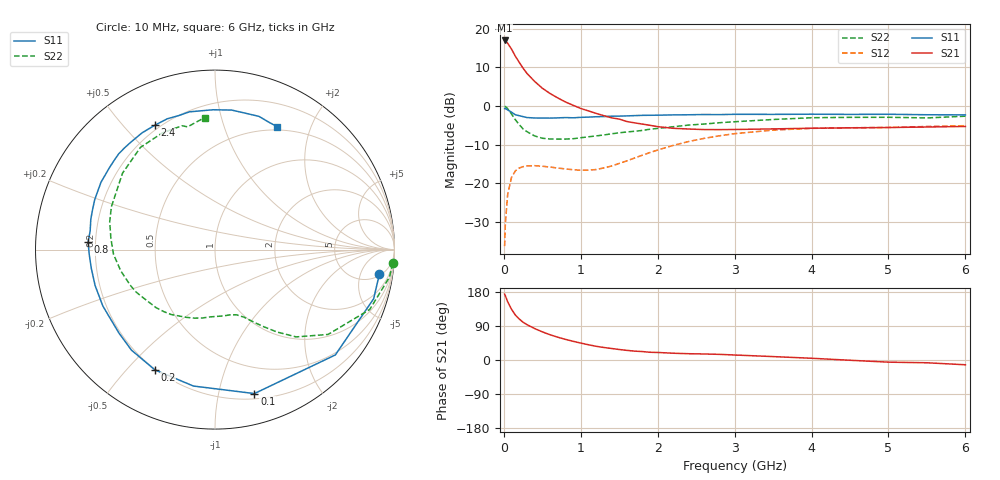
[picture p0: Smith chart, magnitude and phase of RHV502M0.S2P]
! SIEMENS Small Signal Semiconductors
! BFR106
! Si NPN RF Bipolar Junction Transistor in SOT23
! VCE = 0.5 V  IC = 2 mA
! Common Emitter S-Parameters:  August  1996
# GHz  S  MA  R  50
!  f  S11  S21  S12  S22
! GHz  MAG  ANG  MAG  ANG  MAG  ANG  MAG  ANG
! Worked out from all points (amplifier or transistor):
!   36 points, 10 MHz to 6 GHz, reference 50 ohm
!   highest |S21| = 17.0 dB at 10 MHz (marker M1)
!   |S21| within 3 dB of that: start of sweep to 120.3 MHz
!   unconditionally stable (mu >= 1): 737.2 MHz to end of sweep
!   at 250 MHz: K = 0.35, MSG = 12.8 dB, |S12| = -15.7 dB
!   at 1.4 GHz: K = 1.40, MAG = 2.5 dB, |S12| = -15.6 dB
!   at 6 GHz: K = 1.03, MAG = -1.1 dB, |S12| = -5.1 dB
!   S11 on the Smith chart (normalised r, x): 10 MHz: 5, -11; 100 MHz: 0.25, -1.28; 200 MHz: 0.20, -0.60; 800 MHz: 0.17, +0.03; 2.4 GHz: 0.18, +0.61; 6 GHz: 0.46, +1.53
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0.01  0.9259 -8.6  7.087 173.9  0.0152 85.9  0.9929 -4.4
0.02  0.9253 -17.2  6.999 169.3  0.0302 82.7  0.9839 -9.0
0.05  0.891 -41.2  6.503 153.5  0.0716 66.5  0.9242 -21.2
0.1  0.8316 -74.7  5.468 133.9  0.1189 49.7  0.7874 -36.9
0.15  0.7696 -99.0  4.422 118.6  0.144 37.6  0.664 -47.1
0.2  0.749 -116.6  3.688 108.2  0.157 30.3  0.5738 -53.1
0.25  0.7283 -129.7  3.094 99.6  0.1633 24.7  0.5046 -58.0
0.3  0.7088 -139.1  2.653 93.4  0.167 21.4  0.4654 -61.2
0.4  0.6995 -153.3  2.087 83.0  0.1684 16.8  0.4094 -66.8
0.5  0.6974 -163.3  1.703 74.3  0.1654 14.3  0.3819 -71.9
0.6  0.6971 -171.5  1.455 66.7  0.1616 13.6  0.3729 -77.3
0.8  0.7083 176.5  1.129 54.5  0.1527 15.6  0.3724 -89.0
1.1  0.7181 161.6  0.864 40.2  0.1471 26.4  0.3988 -106.8
1.6  0.7444 142.3  0.629 25.4  0.1942 44.8  0.4609 -135.5
2.2  0.767 122.0  0.514 17.9  0.3081 45.1  0.5382 -167.3
2.4  0.7697 115.9  0.503 16.6  0.3461 42.1  0.5659 -177.3
2.8  0.7735 105.2  0.494 14.9  0.4104 34.5  0.6068 165.2
3.5  0.7791 90.8  0.505 9.0  0.4868 20.7  0.6685 140.4
4.5  0.7786 77.1  0.521 -0.7  0.5222 4.4  0.713 114.5
5  0.7816 71.7  0.526 -5.7  0.5271 -1.7  0.7142 104.9
5.5  0.7703 66.9  0.534 -7.3  0.5424 -4.6  0.7006 102.6
6  0.7676 63.1  0.543 -12.6  0.5561 -11.0  0.7379 94.5
